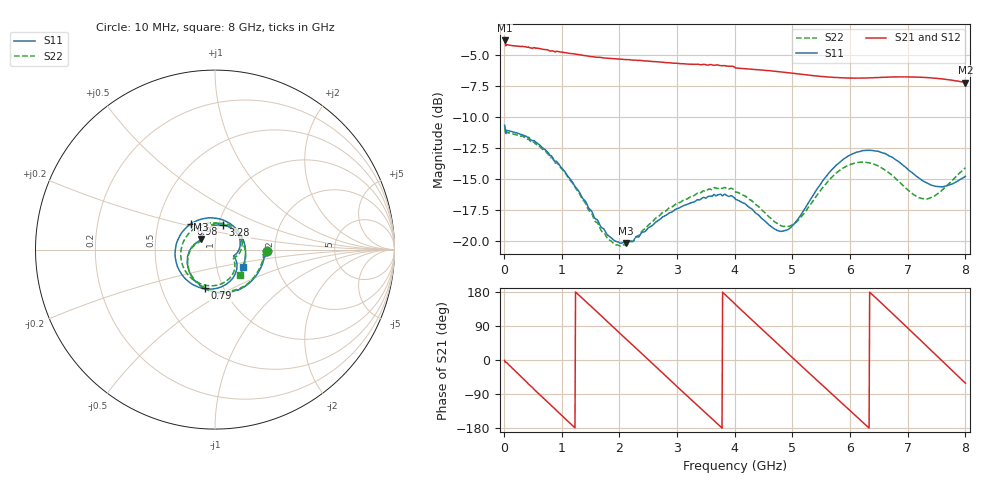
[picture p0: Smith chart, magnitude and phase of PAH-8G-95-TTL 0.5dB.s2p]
! MTS Systemtechnik GmbH
! S-Parameters
! Model: PAH-8G/95-TTL
! Attenuation Step: 0.5dB
! Rohde & Schwarz ZVB8 2Ports - Version 4.11 - 1145.1010k08 SN: 100119
! S2P File Measurements:
! S11 S21 S12 S22
# HZ  S  DB  R  50.00
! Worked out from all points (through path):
!   800 points, 10 MHz to 8 GHz, reference 50 ohm
!   highest |S21| = -3.84 dB at 10 MHz (marker M1); lowest = -7.2 dB at 8 GHz (marker M2)
!   group delay of S21, straight-line fit = 394 ps
!   lowest |S11| = -20.2 dB at 2.12 GHz (marker M3), VSWR 1.22, Z = 42.5 + j5.05 ohm
!   |S11| at or under -10 dB: start of sweep to end of sweep
!   |S22| runs from -20.4 to -10.8 dB; largest |S21 - S12| = 0.0067
!   S11 on the Smith chart (normalised r, x): 10 MHz: 1.82, -0.03; 790 MHz: 0.82, -0.37; 3.28 GHz: 1.05, +0.29; 6.98 GHz: 0.74, +0.22; 8 GHz: 1.34, -0.27
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1e7  -10.69 -1.6  -3.84 -1.2  -3.77 -1.1  -10.83 -1.3
4.3e8  -11.68 -59.2  -4.40 -64.1  -4.39 -64.1  -11.84 -59.2
7.9e8  -13.07 -105.2  -4.68 -115.8  -4.65 -115.8  -13.24 -105.7
1.08e9  -14.61 -141.5  -4.84 -157.6  -4.84 -157.6  -14.66 -141.6
1.35e9  -16.49 -170.6  -5.03 163.9  -5.03 163.9  -16.59 -170.3
1.75e9  -19.20 158.4  -5.25 107.4  -5.26 107.6  -19.47 160.2
2.12e9  -20.22 142.9  -5.38 54.8  -5.39 55.0  -20.37 146.9
2.41e9  -19.31 129.7  -5.48 13.9  -5.46 14.0  -19.15 134.6
2.68e9  -18.35 113.2  -5.58 -24.5  -5.57 -24.3  -18.04 117.5
2.99e9  -17.44 91.4  -5.68 -68.6  -5.68 -68.8  -17.01 95.0
3.28e9  -16.90 71.3  -5.77 -109.4  -5.79 -109.7  -16.39 73.7
3.68e9  -16.39 43.6  -5.82 -165.5  -5.80 -165.1  -15.75 44.0
4.01e9  -16.66 18.7  -6.06 146.7  -6.06 146.6  -16.07 18.2
4.55e9  -18.54 -12.8  -6.27 70.1  -6.29 70.2  -17.88 -16.1
4.95e9  -19.03 -20.3  -6.45 13.4  -6.47 13.3  -18.83 -26.5
5.34e9  -16.49 -35.0  -6.67 -41.3  -6.68 -41.3  -16.92 -38.9
5.87e9  -13.47 -82.2  -6.85 -115.2  -6.88 -115.2  -14.16 -82.4
6.28e9  -12.71 -129.7  -6.87 -172.6  -6.89 -172.6  -13.68 -128.5
6.67e9  -13.14 178.8  -6.80 132.1  -6.80 132.2  -14.51 179.1
6.98e9  -14.14 133.3  -6.78 87.4  -6.78 87.4  -15.81 129.3
7.5e9  -15.62 46.1  -6.89 11.7  -6.89 11.6  -16.27 31.2
8e9  -14.80 -31.9  -7.24 -61.2  -7.24 -61.2  -14.12 -45.0
